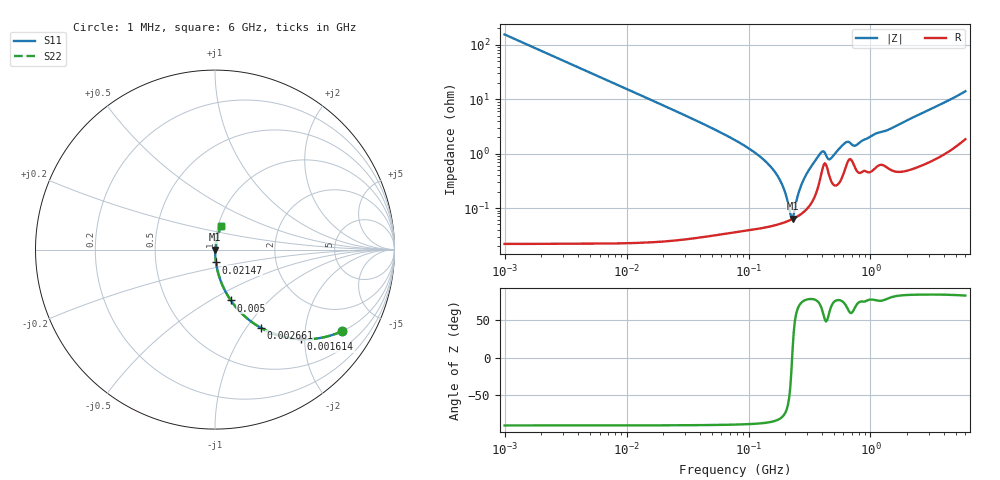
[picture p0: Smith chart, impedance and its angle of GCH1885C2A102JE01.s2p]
!Murata Part Number: GCH1885C2A102JE01
!These Parameters are Measured in Series Mode Connection
!Data Generated on Mar 13, 2026
!  o--ll--o
!Port1  Port2
!  o------o
!Operation Temp=25[degC], DC Bias Voltage=0[V]
!Freq. Start=1000[kHz] Stop=6[GHz] 401[Steps]
# Hz S RI R 50
!Freq.(Hz) S11(Real) S11(Imag) S21(Real) S21(Imag) S12(Real) S12(Imag) S22(Real) S22(Imag)
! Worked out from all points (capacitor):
!   401 points, 1 MHz to 6 GHz, reference 50 ohm
!   read as one part in series: C = 1.02 nF near 1.044 MHz
!   lowest |Z| = 63.9 mohm at 229.8 MHz (marker M1)
!   series resonance near 227.8 MHz, so ESL is about 480 pH
!   S11 on the Smith chart (normalised r, x): 1 MHz: 1.00, -3.11; 1.614 MHz: 1.00, -1.92; 2.661 MHz: 1.00, -1.17; 5 MHz: 1.00, -0.62; 21.47 MHz: 1.00, -0.14; 6 GHz: 1.04, +0.28
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1000000  0.7069 -0.4551  0.2931 0.4551  0.2931 0.4551  0.7069 -0.4551
1613609  0.4809 -0.4995  0.5191 0.4995  0.5191 0.4995  0.4809 -0.4995
2660982  0.2541 -0.4352  0.7459 0.4352  0.7459 0.4352  0.2541 -0.4352
4293785  0.1158 -0.3196  0.8842 0.3196  0.8842 0.3196  0.1158 -0.3196
4999862  0.0881 -0.2831  0.9119 0.2831  0.9119 0.2831  0.0881 -0.2831
1.843659e7  0.00718 -0.083  0.9928 0.083  0.9928 0.083  0.00718 -0.083
2.146833e7  0.00535 -0.0713  0.9946 0.0713  0.9946 0.0713  0.00535 -0.0713
7.745967e7  0.000671 -0.0177  0.9993 0.0177  0.9993 0.0177  0.000671 -0.0177
1.196694e8  0.000504 -0.00944  0.9995 0.00944  0.9995 0.00944  0.000504 -0.00944
1.587717e8  0.000498 -0.0051  0.9995 0.0051  0.9995 0.0051  0.000498 -0.0051
1.889453e8  0.000534 -0.00262  0.9995 0.00262  0.9995 0.00262  0.000534 -0.00262
2.016844e8  0.000558 -0.00171  0.9994 0.00171  0.9994 0.00171  0.000558 -0.00171
2.200158e8  0.0006 -0.00049  0.9994 0.00049  0.9994 0.00049  0.0006 -0.00049
2.297971e8  0.000627 0.000125  0.9994 -0.000125  0.9994 -0.000125  0.000627 0.000125
2.734687e8  0.000799 0.00268  0.9992 -0.00268  0.9992 -0.00268  0.000799 0.00268
3.325952e8  0.00134 0.00604  0.9987 -0.00604  0.9987 -0.00604  0.00134 0.00604
3.958029e8  0.00437 0.00965  0.9956 -0.00965  0.9956 -0.00965  0.00437 0.00965
4.710229e8  0.00336 0.00732  0.9966 -0.00732  0.9966 -0.00732  0.00336 0.00732
6.249308e8  0.00569 0.0149  0.9943 -0.0149  0.9943 -0.0149  0.00569 0.0149
7.600468e8  0.00527 0.0132  0.9947 -0.0132  0.9947 -0.0132  0.00527 0.0132
1.428092e9  0.00592 0.0273  0.9941 -0.0273  0.9941 -0.0273  0.00592 0.0273
6e9  0.0361 0.1318  0.9639 -0.1318  0.9639 -0.1318  0.0361 0.1318
